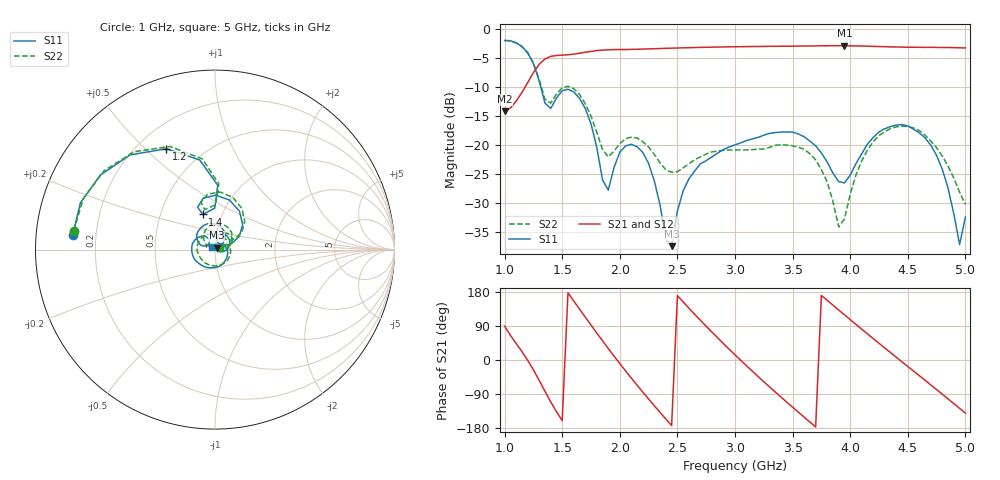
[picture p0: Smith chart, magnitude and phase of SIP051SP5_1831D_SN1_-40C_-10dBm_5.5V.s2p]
# GHz  S  dB  R  50
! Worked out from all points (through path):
!   81 points, 1 GHz to 5 GHz, reference 50 ohm
!   highest |S21| = -2.86 dB at 3.95 GHz (marker M1); lowest = -14.2 dB at 1 GHz (marker M2)
!   lowest |S11| = -37.4 dB at 2.45 GHz (marker M3), VSWR 1.03, Z = 50.9 + j1.05 ohm
!   |S11| at or under -10 dB: 1.314 GHz to end of sweep
!   |S22| runs from -34.1 to -2.0 dB; largest |S21 - S12| = 0.0022
!   S11 on the Smith chart (normalised r, x): 1 GHz: 0.11, +0.05; 1.2 GHz: 0.32, +0.58; 1.4 GHz: 0.81, +0.33; 5 GHz: 0.96, +0.03
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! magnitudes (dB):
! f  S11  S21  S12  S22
! 1 GHz  -2.0  -14.2  -14.2  -2.0
! 1.2 GHz  -4.1  -9.2  -9.2  -4.1
! 1.4 GHz  -13.7  -4.7  -4.7  -12.8
! 1.55 GHz  -10.4  -4.4  -4.4  -9.8
! 1.7 GHz  -13.7  -4.0  -4.0  -12.8
! 1.9 GHz  -27.7  -3.6  -3.6  -22.0
! 2 GHz  -21.2  -3.5  -3.5  -19.7
! 2.1 GHz  -19.8  -3.5  -3.5  -18.6
! 2.25 GHz  -23.1  -3.4  -3.4  -20.3
! 2.35 GHz  -30.3  -3.4  -3.3  -23.0
! 2.45 GHz  -37.4  -3.3  -3.3  -24.6
! 2.6 GHz  -25.8  -3.2  -3.2  -23.2
! 3 GHz  -19.9  -3.1  -3.0  -20.8
! 3.7 GHz  -20.1  -2.9  -2.9  -22.5
! 3.9 GHz  -26.3  -2.9  -2.9  -34.1
! 3.95 GHz  -26.5  -2.9  -2.9  -32.7
! 4.1 GHz  -21.5  -2.9  -2.9  -22.7
! 4.35 GHz  -16.8  -3.1  -3.1  -17.1
! 4.7 GHz  -20.0  -3.1  -3.1  -19.3
! 4.85 GHz  -27.4  -3.2  -3.2  -23.6
! 4.95 GHz  -37.1  -3.2  -3.2  -28.1
! 5 GHz  -32.3  -3.3  -3.3  -30.2
